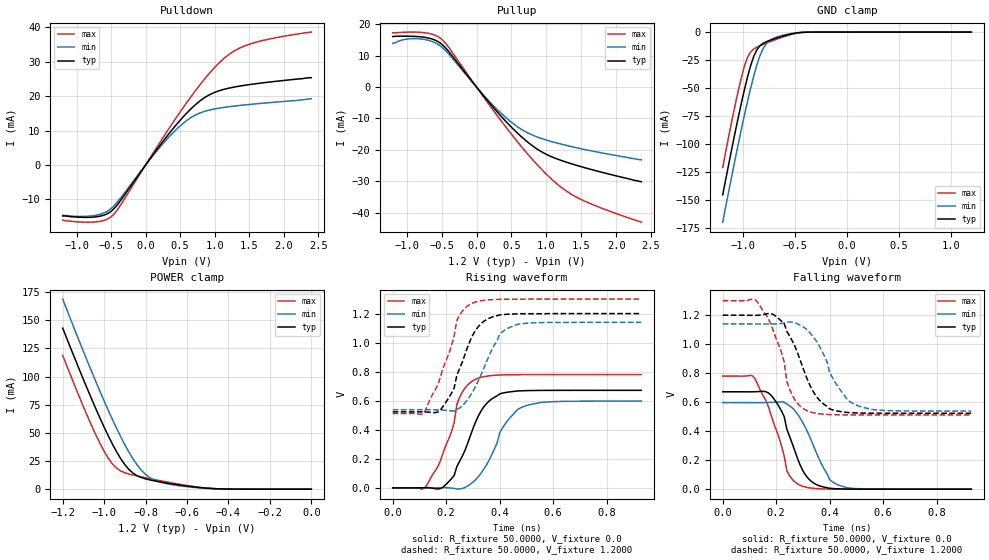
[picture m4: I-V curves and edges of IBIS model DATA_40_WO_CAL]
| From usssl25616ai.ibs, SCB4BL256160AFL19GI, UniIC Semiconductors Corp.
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|   Model DATA_40_WO_CAL
[Model]  DATA_40_WO_CAL
Model_type I/O
Polarity   Non-Inverting
Enable   Active-High
Vinl =   0.3800V
Vinh =   0.8200V
Vmeas =  0.6000V
Cref =   5.0000pF
Rref =   50.0000
Vref =   0.6000V
C_comp   1.7430pF   1.7110pF   1.7640pF
[Temperature Range]   25.0000   85.0000   -40.0000
[Voltage Range]   1.2000V   1.1400V   1.3000V
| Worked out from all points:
|   slope of the pulldown table from 0 to 0.18 V, typ, clamps not added: 36.2 ohm
|   slope of the pullup table from 0 to 0.18 V, typ, clamps not added: 36.7 ohm
|   GND clamp passes 1 mA (typ) near -0.50 V on its own axis
|   POWER clamp passes 1 mA (typ) near -0.51 V on its own axis
|   rising waveform, R_fixture 50.0000, V_fixture 0.0: 20-80 % time 95.4ps typ, 99.1ps min, 79.3ps max; typ from 0 V to 0.672 V
|   rising waveform, R_fixture 50.0000, V_fixture 1.2000: 20-80 % time 81.5ps typ, 93.7ps min, 81.3ps max; typ from 0.523 V to 1.2 V
|   falling waveform, R_fixture 50.0000, V_fixture 0.0: 20-80 % time 77.9ps typ, 92.4ps min, 79.3ps max; typ from 0.672 V to 0 V
|   falling waveform, R_fixture 50.0000, V_fixture 1.2000: 20-80 % time 96.1ps typ, 100ps min, 75.8ps max; typ from 1.2 V to 0.523 V
[Pulldown]
|Voltage   I(typ)   I(min)   I(max)
-1.2V     -14.8mA    -14.6mA    -16mA
-720mV    -15.06mA   -14.6mA    -16.52mA
-480mV    -13.11mA   -12.3mA    -14.71mA
-360mV    -10.25mA   -9.502mA   -11.57mA
200mV     5.517mA    5.003mA    6.349mA
520mV     13.45mA    11.72mA    16mA
680mV     16.78mA    14.09mA    20.49mA
840mV     19.41mA    15.53mA    24.66mA
1.2V      22.33mA    16.94mA    32.04mA
1.36V     22.95mA    17.32mA    33.99mA
1.6V      23.66mA    17.8mA     35.73mA
2.4V      25.4mA     19.3mA     38.66mA
[Pullup]
|Voltage   I(typ)   I(min)   I(max)
-1.2V     16.1mA     13.9mA     17.3mA
-1.04V    16.21mA    15.14mA    17.47mA
-840mV    16.09mA    15.42mA    17.5mA
-640mV    15.36mA    14.57mA    16.89mA
-520mV    14.05mA    13.16mA    15.63mA
-400mV    11.39mA    10.58mA    12.74mA
320mV     -8.514mA   -7.675mA   -9.807mA
600mV     -14.97mA   -12.85mA   -17.81mA
840mV     -19.35mA   -15.66mA   -24.06mA
1.12V     -22.63mA   -17.66mA   -30.27mA
1.4V      -24.74mA   -19.2mA    -34.72mA
2.36V     -30.2mA    -23.2mA    -43.09mA
[GND_clamp]
|Voltage   I(typ)   I(min)   I(max)
-1.2V     -145.3mA   -169.7mA   -120.8mA
-1.11V    -103.1mA   -127.3mA   -78.51mA
-1.05V    -76.2mA    -100.1mA   -52.43mA
-990mV    -51.2mA    -74mA      -30.39mA
-960mV    -39.9mA    -61.63mA   -22.48mA
-900mV    -21.67mA   -39mA      -15mA
-870mV    -15.78mA   -29.25mA   -13.45mA
-810mV    -10.04mA   -14.72mA   -11.07mA
-750mV    -7.557mA   -7.71mA    -8.865mA
-600mV    -3.111mA   -2.463mA   -3.804mA
-420mV    -215.4uA   -156.1uA   -235uA
1.2V      1.597nA    5.589nA    1.463nA
[POWER_clamp]
|Voltage   I(typ)   I(min)   I(max)
-1.2V     143mA      168.8mA    118.7mA
-1.06V    79.88mA    104.3mA    56.26mA
-1.02V    63.08mA    86.79mA    40.63mA
-980mV    47.32mA    69.97mA    27.48mA
-940mV    33.2mA     54.05mA    18.67mA
-880mV    17.43mA    32.78mA    13.45mA
-840mV    11.87mA    21.34mA    11.69mA
-800mV    9.133mA    13.1mA     10.12mA
-720mV    6.135mA    5.731mA    7.166mA
-560mV    1.838mA    1.456mA    2.161mA
-420mV    156.9uA    132.7uA    153uA
0V        1.597nA    1.927nA    2.16nA
[Ramp]
| variable   typ   min   max
dV/dt_r  0.4030/90.3786p   0.3584/0.1015n   0.4679/83.0159p
dV/dt_f  0.4060/89.3830p   0.3611/0.1028n   0.4729/79.8092p
R_load = 50.0000
[Rising Waveform]
R_fixture= 50.0000
V_fixture= 0.0
V_fixture_min= 0.0
V_fixture_max= 0.0
|time   V(typ)   V(min)   V(max)
0s        0V         0V         0V
120ps     1.042mV    167.9uV    -141.5uV
170ps     -7.981mV   991.8uV    149.9mV
230ps     85.52mV    -3.562mV   450.3mV
250ps     182mV      -7.996mV   621.6mV
310ps     453.7mV    55.7mV     747.5mV
370ps     611.7mV    226.4mV    773.3mV
410ps     651.9mV    410.7mV    778.1mV
480ps     668.3mV    552.4mV    779.6mV
930ps     671.6mV    597.3mV    779.8mV
[Rising Waveform]
R_fixture= 50.0000
V_fixture= 1.2000
V_fixture_min= 1.1400
V_fixture_max= 1.3000
|time   V(typ)   V(min)   V(max)
0s        523.4mV    538.2mV    511.9mV
110ps     523.3mV    538.5mV    506.1mV
180ps     539.9mV    536mV      774.1mV
230ps     688.5mV    529.9mV    1.047V
240ps     775.7mV    538.8mV    1.153V
300ps     1.054V     664.9mV    1.273V
340ps     1.146V     820.6mV    1.291V
400ps     1.191V     1.058V     1.298V
440ps     1.196V     1.107V     1.299V
930ps     1.2V       1.14V      1.3V
[Falling Waveform]
R_fixture= 50.0000
V_fixture= 0.0
V_fixture_min= 0.0
V_fixture_max= 0.0
|time   V(typ)   V(min)   V(max)
0s        671.6mV    597.3mV    779.8mV
120ps     671.8mV    597mV      763.9mV
170ps     664.7mV    597.7mV    574.8mV
210ps     571.5mV    601.3mV    359.3mV
240ps     413.2mV    586.9mV    126.3mV
290ps     165mV      489.4mV    26.55mV
340ps     42.49mV    297mV      5.485mV
400ps     5.96mV     66.29mV    598.4uV
430ps     2.556mV    31.06mV    231uV
930ps     0V         0V         0V
[Falling Waveform]
R_fixture= 50.0000
V_fixture= 1.2000
V_fixture_min= 1.1400
V_fixture_max= 1.3000
|time   V(typ)   V(min)   V(max)
0s        1.2V       1.14V      1.3V
130ps     1.199V     1.139V     1.291V
180ps     1.211V     1.139V     1.139V
230ps     1.141V     1.145V     877.9mV
240ps     1.089V     1.151V     743.4mV
260ps     1.023V     1.153V     648.5mV
310ps     787.6mV    1.108V     546.1mV
400ps     553.8mV    805.4mV    513.9mV
490ps     526.4mV    588.2mV    512mV
930ps     523.4mV    538.2mV    511.9mV
